TYPE ST_AxisPara :
STRUCT
	TargetPos:LREAL:=10;(*NC轴绝对定位位置*)
	MoveVelo:LREAL:=10;(*NC轴绝对定位的速度*)
	JogVelo:LREAL:=10;(*NC轴点动速度*)
	RefPos:LREAL;(*NC轴寻参完成时的原点位置*)
	SetPosition:LREAL;

	rOverride:LREAL:=100.0;
	rMoveSuperDistance:LREAL:=10;
	HomingMode		:BYTE	:=1;(*0: 标准寻参 1:Johnson寻参;  2: Swen寻参*)
END_STRUCT
END_TYPE
